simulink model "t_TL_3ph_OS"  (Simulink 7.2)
settings: Solver=ode3  StartTime=0.0  StopTime=0.2  FixedStep=1e-6  RelTol=1e-3

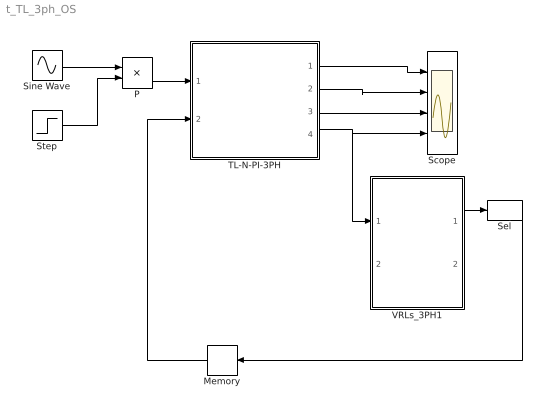
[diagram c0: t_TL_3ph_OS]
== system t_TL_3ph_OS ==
  Memory : Memory  Orientation=left
  P : Product
  Scope : Scope  NumInputPorts=4
  Sel : Selector  InputPortWidth=3  IndexOptions=Index vector (dialog)  Indices=[1 2]  OutputSizes=1
  Sine Wave : Sin  Amplitude=230000*sqrt(2/3)  Frequency=50*2*pi  Phase="[0  -2*pi/3  -4*pi/3]"  SampleTime=0
  Step : Step  Time=0.024*1  SampleTime=0
  TL-N-PI-3PH : Subsystem  mask(3-Phase TL N-PI-Sections){R=0.01273, L=0.9337e-3, C=12.74e-9, TL=100, N=5, RS=1e-3, LS=1e-3}
      mask prompts: R "R/km"; L "L/km"; C "C/km"; TL "Length[km]"; N "N_Sections"
      mask help: 3 Phase trans. Line as N-PI-Sections Input Vector: u[0,1,2]=Input Voltages u[3.4]=Load Currents Output Vector: y[0,1,2]=Input Currents y[3,4,5]=Output Currents y[6,7,8]=Input Voltages y[9,10,11]=Output Voltages PArameter Vector: p[0]= TL-Resistance R/km p[1]= TL-Inductane L/km p[2]= TL-Capacitance C/km p[3]= TL-Length [km] p[4]= Number of PI-Sections N p[5]= Source-Input Resistance R
  VRLs_3PH1 : Subsystem  mask(VRLs_3PH_OS){R=1, L=1e-3, RLp=1e6}
      mask prompts: R "Output Resistance"; L "Output Inductance"; RLp "Ind. Parallel Res"
      mask help: Open source 3 Phase VRL_Series Input Vector: u[0,1,2]= Vs1, Vs2, Vs3, Source Voltages u[3,4,5]= E1, E2, E3, Load Voltages Output Vector: y[0,1,2]=IL1, IL2, IL3 Load currents y[3,4,5]=VL1, VL2, VL3 Inductance Voltages Parameter Vector: p[0]=R p[1]=L
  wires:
  Sine Wave/1 -> P/1
  P/1 -> TL-N-PI-3PH/1(VS_ABC)
  Step/1 -> P/2
  TL-N-PI-3PH/4(Vabc) -> Scope/4, VRLs_3PH1/1(V123)
  VRLs_3PH1/1(iL123) -> Sel/1
  Memory/1 -> TL-N-PI-3PH/2(IL12)
  TL-N-PI-3PH/1(IABC) -> Scope/1
  TL-N-PI-3PH/3(VABC) -> Scope/3
  TL-N-PI-3PH/2(Iabc) -> Scope/2
  Sel/1 -> Memory/1

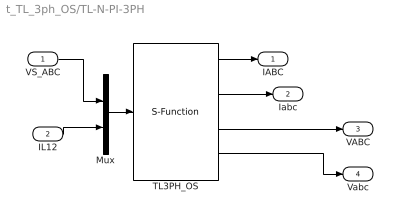
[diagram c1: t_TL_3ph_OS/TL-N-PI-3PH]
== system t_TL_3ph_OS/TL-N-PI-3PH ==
  VS_ABC : Inport  OutDataType=sfix(16)  OutScaling=2^0
  IL12 : Inport  Port=2  OutDataType=sfix(16)  OutScaling=2^0
  Mux : Mux  Inputs="[3  2]"
  TL3PH_OS : S-Function  FunctionName=s_TL_N_PI_3PH_OS  Parameters=[R L C TL N RS LS ]  EnableBusSupport=off
  IABC : Outport  OutDataType=sfix(16)  OutScaling=2^0
  Iabc : Outport  Port=2  OutDataType=sfix(16)  OutScaling=2^0
  VABC : Outport  Port=3  OutDataType=sfix(16)  OutScaling=2^0
  Vabc : Outport  Port=4  OutDataType=sfix(16)  OutScaling=2^0
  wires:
  TL3PH_OS/4 -> Vabc/1
  Mux/1 -> TL3PH_OS/1
  VS_ABC/1 -> Mux/1
  IL12/1 -> Mux/2
  TL3PH_OS/1 -> IABC/1
  TL3PH_OS/3 -> VABC/1
  TL3PH_OS/2 -> Iabc/1

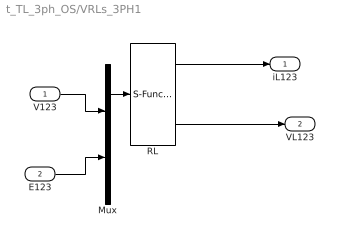
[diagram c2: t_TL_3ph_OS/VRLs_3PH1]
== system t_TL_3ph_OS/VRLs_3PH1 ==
  V123 : Inport
  E123 : Inport  Port=2
  Mux : Mux  Inputs="[3  3]"
  RL : S-Function  FunctionName=s_VRLs_3PH_OS  Parameters=[R, L, RLp]  EnableBusSupport=off
  iL123 : Outport
  VL123 : Outport  Port=2
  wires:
  RL/2 -> VL123/1
  RL/1 -> iL123/1
  Mux/1 -> RL/1
  V123/1 -> Mux/1
  E123/1 -> Mux/2
